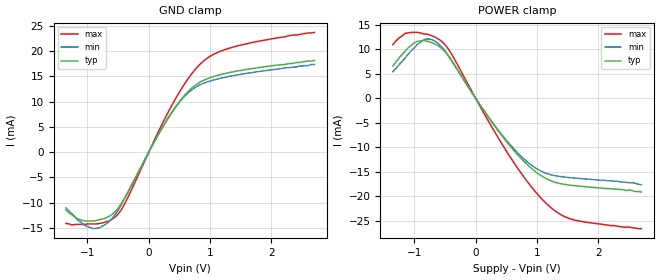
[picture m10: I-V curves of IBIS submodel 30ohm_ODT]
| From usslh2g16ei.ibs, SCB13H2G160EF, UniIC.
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| SUBMODEL 30ohm_ODT
[Submodel]   30ohm_ODT
Submodel_type  Dynamic_clamp
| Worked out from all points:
|   GND clamp passes 1 mA (typ) near -0.04 V on its own axis
|   POWER clamp passes 1 mA (typ) near -0.05 V on its own axis
[GND Clamp]
|Voltage   I(typ)   I(min)   I(max)
-1.35V    -11.4mA    -11mA      -14.06mA
-1.15V    -13.2mA    -13.5mA    -14.27mA
-900mV    -13.6mA    -15.1mA    -14.17mA
-650mV    -12.69mA   -13.72mA   -13.59mA
-500mV    -11.08mA   -11.45mA   -12.23mA
-400mV    -9.181mA   -9.306mA   -10.36mA
100mV     2.276mA    2.274mA    2.618mA
400mV     8.316mA    8.244mA    9.773mA
650mV     12.08mA    11.81mA    14.66mA
900mV     14.23mA    13.63mA    18.07mA
1.45V     16.04mA    15.27mA    21mA
2.7V      18.1mA     17.3mA     23.65mA
[POWER Clamp]
|Voltage   I(typ)   I(min)   I(max)
-1.35V    6.6mA      5.4mA      10.94mA
-1.15V    9.6mA      8.2mA      13.23mA
-1V       11.3mA     10.3mA     13.44mA
-850mV    11.8mA     11.9mA     13.12mA
-700mV    11.28mA    11.9mA     12.69mA
-400mV    7.848mA    7.858mA    9.19mA
150mV     -2.816mA   -2.766mA   -3.376mA
550mV     -9.562mA   -9.285mA   -11.72mA
900mV     -14.18mA   -13.52mA   -17.91mA
1.2V      -16.67mA   -15.49mA   -21.99mA
1.6V      -17.79mA   -16.23mA   -24.77mA
2.7V      -19.1mA    -17.6mA    -26.56mA
